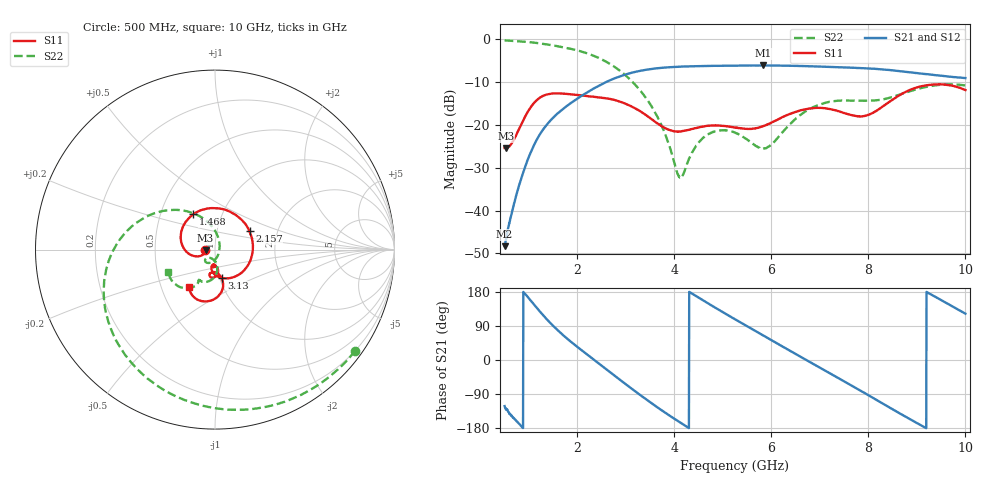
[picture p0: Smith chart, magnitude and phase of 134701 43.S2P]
!  2-Port S-parameters saved by WinCal
! VAR MeasName=S-Parameters (CALIBRATED_DATA) read from VNA (N5242A)
! VAR MeasDate=2013-7-3 16:38:00
! VAR NAME=134701 43
! VAR FILENAME=134701 43.S2P
! VAR DATE=2013-7-3 16:38:00
! VAR PHYS_PORTS=1,2
# Hz S MA R 50
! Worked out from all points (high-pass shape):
!   1601 points, 500 MHz to 10 GHz, reference 50 ohm
!   highest |S21| = -6.16 dB at 5.832 GHz (marker M1); lowest = -48.3 dB at 500 MHz (marker M2)
!   |S21| within 3 dB of the highest: 2.77 GHz to end of sweep
!   lowest |S11| = -25.5 dB at 523.8 MHz (marker M3), VSWR 1.11, Z = 45 - j0.382 ohm
!   |S11| at or under -10 dB: start of sweep to end of sweep
!   |S22| runs from -32.4 to -0.3 dB; largest |S21 - S12| = 0.0018
!   S11 on the Smith chart (normalised r, x): 500 MHz: 0.90, -0.00; 1.468 GHz: 0.73, +0.30; 2.157 GHz: 1.44, +0.31; 3.13 GHz: 1.02, -0.33; 10 GHz: 0.69, -0.31
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5e8  0.05355 -177.4  0.00384 -121.8  0.003879 -125.1  0.9631 -35.9
5.2375e8  0.05308 -175.4  0.004446 -127.5  0.004438 -128.9  0.9617 -37.6
7.375e8  0.07557 -157.0  0.01489 -159.5  0.01495 -160.1  0.9479 -52.7
9.75e8  0.1412 -168.5  0.03909 166.6  0.03905 166.2  0.925 -69.5
1.224375e9  0.2067 157.4  0.07699 128.3  0.07688 128.2  0.8906 -87.1
1.467812e9  0.2308 121.3  0.1158 94.4  0.1157 94.3  0.8485 -103.7
2.085312e9  0.2204 37.3  0.2174 25.9  0.2168 25.9  0.7146 -146.6
2.156562e9  0.2179 28.1  0.2306 18.8  0.2302 18.8  0.6949 -151.7
2.66125e9  0.2008 -32.0  0.3281 -30.9  0.3282 -30.8  0.5171 171.0
3.130312e9  0.1625 -76.7  0.4058 -76.7  0.4062 -76.6  0.3188 136.0
3.670625e9  0.102 -101.3  0.4583 -126.7  0.4579 -126.7  0.1179 94.1
4.121875e9  0.08342 -93.7  0.4759 -165.1  0.4762 -165.2  0.02398 -9.2
4.626562e9  0.0962 -92.8  0.4847 154.7  0.4847 154.6  0.07321 -105.3
5.25e9  0.09313 -98.0  0.4896 107.5  0.4897 107.5  0.0811 -132.9
5.831875e9  0.09647 -85.2  0.492 64.7  0.4919 64.7  0.05271 -112.8
6.354375e9  0.132 -83.1  0.4883 26.5  0.4892 26.5  0.09817 -82.4
6.835312e9  0.1558 -92.8  0.4814 -8.4  0.4815 -8.4  0.1584 -92.7
7.678438e9  0.1287 -98.7  0.4624 -69.4  0.4632 -69.5  0.1913 -115.7
7.993125e9  0.1306 -85.6  0.4544 -92.3  0.4544 -92.4  0.1911 -117.9
8.420625e9  0.183 -76.3  0.4362 -124.3  0.4355 -124.3  0.2053 -117.2
9.156875e9  0.2863 -95.3  0.3916 -177.5  0.392 -177.5  0.2738 -128.1
1e10  0.2543 -124.5  0.351 122.3  0.351 122.2  0.2876 -154.7
